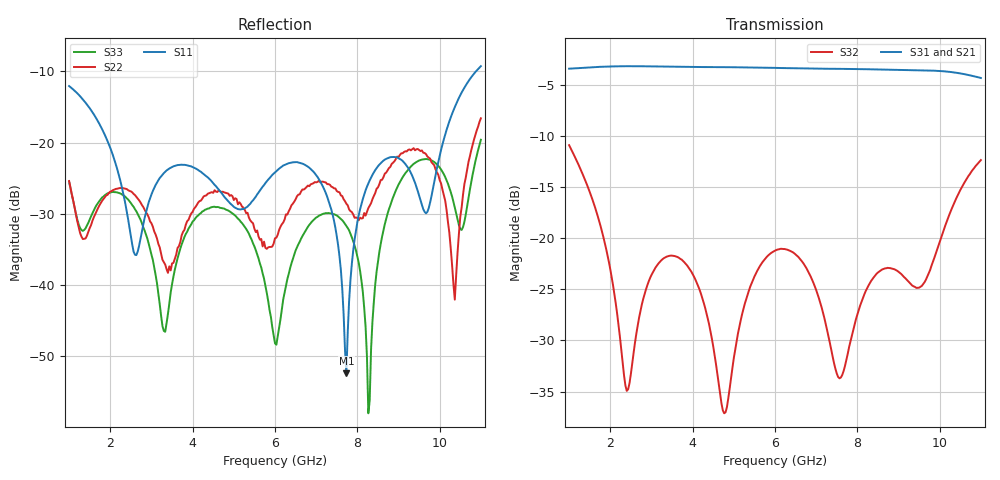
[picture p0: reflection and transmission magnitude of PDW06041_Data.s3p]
# GHz S DB R 50.00000
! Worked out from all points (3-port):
!   301 points, 1 GHz to 11 GHz, reference 50 ohm
!   strongest paths, dB at 1 GHz, 3.5 GHz, 6 GHz, 8.5 GHz, 11 GHz:
!     S31: -3.4, -3.2, -3.4, -3.5, -4.3
!     S21: -3.4, -3.2, -3.4, -3.6, -4.5
!     S32: -10.9, -21.7, -21.2, -23.4, -12.4
!   lowest |S11| = -52.4 dB at 7.733 GHz (marker M1), VSWR 1.00, Z = 49.8 - j0.0467 ohm
!   |S11| at or under -10 dB: start of sweep to 10.88 GHz
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1  -12.06 126.7  -3.43 -69.1  -3.44 -68.7
   -3.43 -69.1  -25.40 15.5  -10.91 -93.9
   -3.43 -68.8  -10.91 -93.9  -25.56 13.7
2.4  -29.70 78.0  -3.18 -169.4  -3.20 -168.6
     -3.18 -169.4  -26.54 110.7  -34.93 -109.9
     -3.19 -168.6  -34.94 -110.0  -27.83 121.2
3.8  -23.13 152.0  -3.26 89.3  -3.26 90.4
     -3.26 89.2  -32.28 138.4  -22.35 -121.9
     -3.26 90.4  -22.37 -121.8  -33.28 163.4
6  -24.19 177.7  -3.36 -72.6  -3.36 -71.0
   -3.37 -72.7  -33.44 95.6  -21.24 -119.0
   -3.36 -71.0  -21.23 -119.1  -48.21 47.8
7.266667  -27.60 118.5  -3.45 -167.9  -3.44 -165.9
          -3.45 -168.0  -25.84 56.0  -29.03 173.5
          -3.44 -165.9  -29.02 173.5  -29.93 27.7
7.733333  -52.41 -168.7  -3.47 156.3  -3.46 158.6
          -3.47 156.2  -28.60 44.6  -31.90 -129.9
          -3.46 158.6  -31.90 -130.0  -31.69 -11.4
8.266667  -25.74 -127.5  -3.52 115.0  -3.49 117.4
          -3.52 115.0  -29.21 83.9  -24.67 -132.1
          -3.49 117.4  -24.67 -132.1  -58.04 -11.9
8.933333  -22.06 -165.6  -3.59 62.9  -3.55 65.5
          -3.60 62.9  -22.33 69.9  -23.13 -162.6
          -3.55 65.5  -23.12 -162.6  -26.75 61.8
10.36667  -15.02 -120.7  -3.87 -53.0  -3.81 -50.2
          -3.88 -53.1  -42.07 58.9  -16.42 -160.4
          -3.81 -50.3  -16.42 -160.3  -29.16 -90.1
11  -9.27 -164.0  -4.40 -104.9  -4.35 -102.2
    -4.46 -105.0  -16.59 84.7  -12.43 162.1
    -4.34 -102.2  -12.37 162.2  -19.61 93.2
